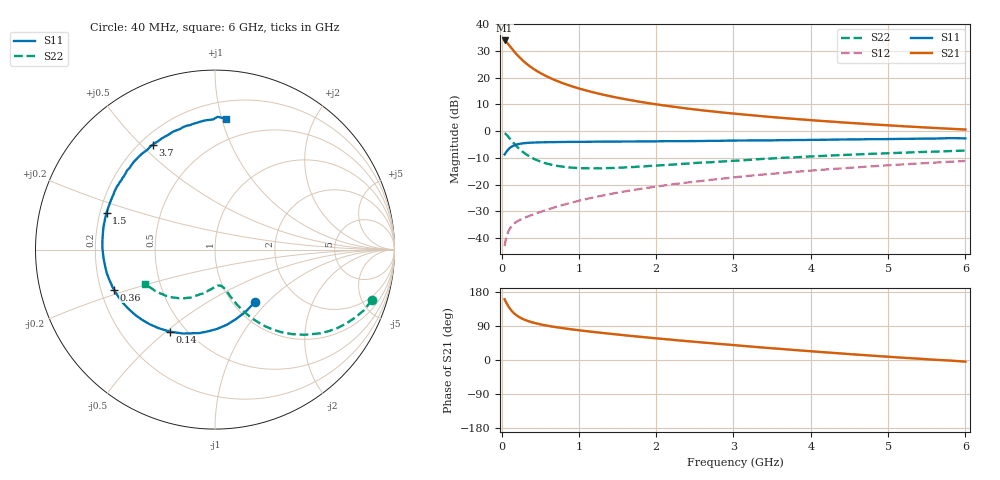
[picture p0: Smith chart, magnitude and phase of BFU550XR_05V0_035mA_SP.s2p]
! Filename:  P:\Prog\Test\Noise\ATS_data\Testdata_Net\03 Spar\BFU550XR_APG2013_45_C05_05p0V_035mA_SP_CM01_D.s2p
! Date/Time: Tue 06/Aug/2013 14:38:16
! BFU550XR_APG2013_45_C05_05p0V_25to35mA_SP_CM01_Bias2_R.s2p
! MDIF S-parameter v. bias file
! BFU550XR_APG2013_45_C05_05p0V_25to35mA_SP_CM01
! Date/time Mon Aug 05 16:56:59 2013
! VAR V_out= 5.0000
! VAR I_out= 35.0000
! VAR V_in= 0.8310
! VAR I_in= 0.3957
! Device data file deembeded for feedlines and parallel
! Original file: \03 Spar\BFU550XR_APG2013_45_C05_05p0V_035mA_SP_CM01_R.s2p
! Feed-files: PR006V01_02082013_Feed1.s2p, PR006V01_02082013_Feed2.s2p
! Parallel-file: PR006V01_02082013_Par.s2p
# MHz S MA R 50
!  Freq-MHz  S11-mag  S11-arg  S21-mag  S21-arg  S12-mag  S12-arg  S22-mag  S22-arg
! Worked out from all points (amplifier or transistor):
!   98 points, 40 MHz to 6 GHz, reference 50 ohm
!   highest |S21| = 33.9 dB at 40 MHz (marker M1)
!   |S21| within 3 dB of that: start of sweep to 132.3 MHz
!   unconditionally stable (mu >= 1): 1.036 GHz to 2.923 GHz
!   at 300 MHz: K = 0.60, MSG = 29.1 dB, |S12| = -32.4 dB
!   at 1.6 GHz: K = 1.04, MAG = 16.1 dB, |S12| = -22.5 dB
!   at 6 GHz: K = 0.83, MSG = 5.9 dB, |S12| = -11.2 dB
!   S11 on the Smith chart (normalised r, x): 40 MHz: 1.26, -0.85; 140 MHz: 0.41, -0.51; 360 MHz: 0.25, -0.18; 1.5 GHz: 0.23, +0.16; 3.7 GHz: 0.25, +0.54; 6 GHz: 0.33, +1.03
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40  0.3668 -52.6  49.62 160.4  0.007054 75.5  0.9179 -17.8
50  0.3846 -63.2  48.05 155.5  0.008622 72.7  0.8974 -22.0
80  0.4419 -88.4  43.47 144.5  0.01238 64.8  0.8088 -32.8
100  0.4733 -100.7  40.11 138.1  0.01439 60.8  0.7468 -38.7
120  0.5004 -110.9  36.96 132.5  0.01597 57.7  0.6886 -43.6
140  0.522 -118.8  34.03 127.8  0.01732 55.4  0.636 -47.7
160  0.5387 -125.6  31.29 123.7  0.0185 53.8  0.5903 -51.2
180  0.5528 -131.2  28.95 120.2  0.01952 52.4  0.5481 -54.2
220  0.5733 -140.1  25.07 114.3  0.02117 51.1  0.4795 -58.7
280  0.5921 -149.7  20.64 107.8  0.02337 50.8  0.4043 -63.5
360  0.606 -158.4  16.59 101.7  0.02601 51.9  0.3379 -67.7
480  0.6161 -167.2  12.74 95.2  0.03009 54.4  0.2784 -71.6
650  0.6229 -175.5  9.55 88.5  0.03608 57.9  0.2346 -75.1
850  0.6285 177.4  7.372 82.4  0.04377 60.6  0.2109 -78.8
1050  0.631 171.7  5.99 77.3  0.05183 62.4  0.2027 -81.6
1500  0.6384 161.1  4.216 67.2  0.07056 63.6  0.2069 -89.2
2050  0.6468 150.2  3.093 56.3  0.09377 62.7  0.2297 -98.2
3100  0.6675 130.8  2.066 37.6  0.1411 57.9  0.2833 -113.6
3700  0.6792 120.7  1.732 27.8  0.1684 53.7  0.3205 -122.1
4100  0.6885 114.0  1.564 21.5  0.187 50.6  0.3409 -127.7
5200  0.7168 96.7  1.232 5.9  0.2388 41.6  0.3955 -142.7
6000  0.7325 85.4  1.072 -4.3  0.2765 34.2  0.4326 -153.7
